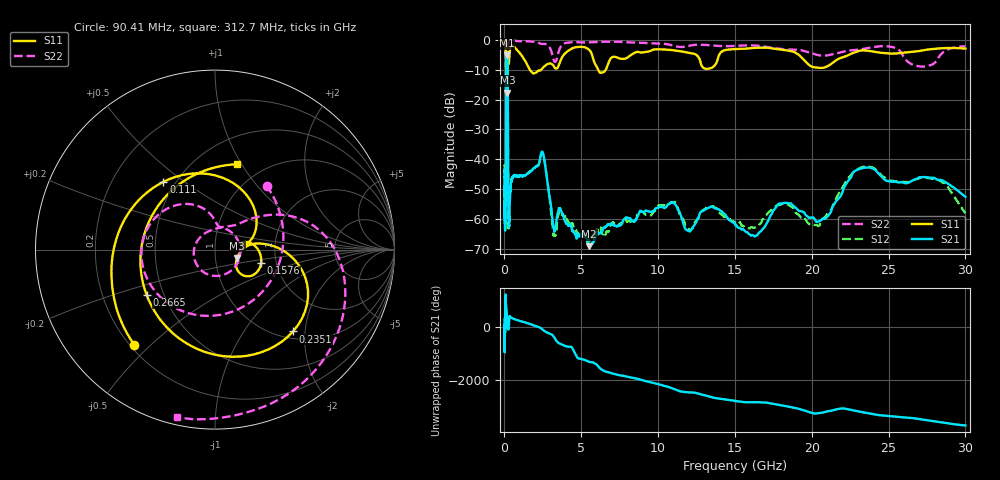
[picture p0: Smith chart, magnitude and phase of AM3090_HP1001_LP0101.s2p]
! Date/Time: Thu, Feb 28, 2019 2:03 PM
! Network Analyzer: Agilent Technologies E8364B Rev: A.07.50.67
! Sweep from 0.010 to 30.000 GHz, 1601 Points, Sweep Type: LOG
! Power Supply: 5.023 V, 0.002 A
# Hz S DB R 50
!freq MagS11 AngS11 MagS21 AngS21 MagS12 AngS12 MagS22 AngS22
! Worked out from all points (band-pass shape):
!   1601 points, 10 MHz to 30 GHz, reference 50 ohm
!   highest |S21| = -5.12 dB at 159.9 MHz (marker M1); lowest = -69.1 dB at 5.501 GHz (marker M2)
!   |S21| within 3 dB of the highest: 123.9 MHz to 204.8 MHz (80.9 MHz wide, 49.2 % of centre)
!   lowest |S11| = -17.6 dB at 191.5 MHz (marker M3), VSWR 1.30, Z = 63.7 - j6.03 ohm
!   |S11| at or under -10 dB: 120.6 MHz to 212.2 MHz (91.54 MHz wide, 55 % of centre); 1.657 GHz to 2.378 GHz (721.3 MHz wide, 35.8 % of centre); 6.099 GHz to 6.59 GHz (491.4 MHz wide, 7.74 % of centre)
!   |S22| runs from -19.4 to -0.2 dB; largest |S21 - S12| = 0.013
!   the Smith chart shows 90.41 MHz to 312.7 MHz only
!   S11 on the Smith chart (normalised r, x): 90.41 MHz: 0.22, -0.44; 111 MHz: 0.43, +0.42; 157.6 MHz: 1.66, -0.27; 235.1 MHz: 1.14, -1.73; 266.5 MHz: 0.40, -0.26; 312.7 MHz: 0.76, +0.96
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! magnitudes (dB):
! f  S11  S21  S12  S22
! 10 MHz  -0.3  -43.6  -46.3  -0.6
! 38.04 MHz  -0.5  -61.1  -59.7  -1.4
! 90.41 MHz  -3.2  -49.5  -49.7  -6.8
! 111 MHz  -6.5  -19.3  -19.3  -7.8
! 144.7 MHz  -13.3  -5.3  -5.3  -17.5
! 157.6 MHz  -11.5  -5.1  -5.1  -16.7
! 159.9 MHz  -11.4  -5.1  -5.1  -16.6
! 191.5 MHz  -17.6  -6.1  -6.1  -19.3
! 214.9 MHz  -9.1  -12.8  -12.7  -11.5
! 235.1 MHz  -4.0  -39.6  -40.6  -2.6
! 266.5 MHz  -6.8  -59.0  -61.4  -0.8
! 312.7 MHz  -6.2  -60.7  -59.3  -0.4
! 550.5 MHz  -2.0  -46.1  -45.6  -0.2
! 2.084 GHz  -10.8  -42.3  -42.3  -0.7
! 2.533 GHz  -9.1  -38.4  -38.5  -1.3
! 3.253 GHz  -9.2  -64.3  -65.5  -7.2
! 5.501 GHz  -3.2  -69.1  -67.5  -0.8
! 7.926 GHz  -6.1  -59.6  -60.6  -0.7
! 16.29 GHz  -2.6  -65.9  -62.9  -1.8
! 20.41 GHz  -9.3  -61.0  -62.4  -5.1
! 23.48 GHz  -3.5  -42.8  -42.4  -2.9
! 30 GHz  -2.8  -52.6  -58.1  -2.2
